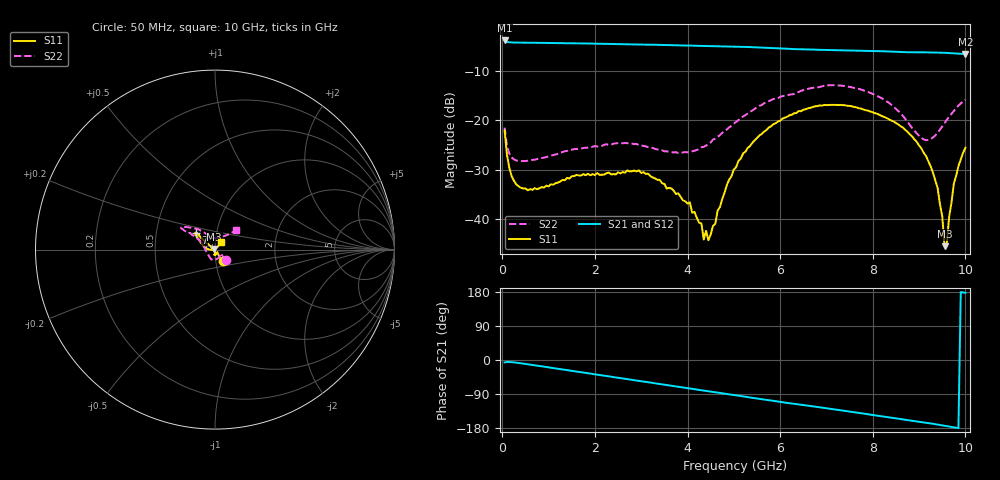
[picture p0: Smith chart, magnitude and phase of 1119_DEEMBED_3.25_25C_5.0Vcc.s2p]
!Hittite Microwave Corp.
!Digital Attenuator/PhaseShifter Rev 1.4.0
!Filename: C:\DATA\DATA\1119_DEEMBED_3.25_25C_5.0Vcc.s2p
!VNA ID: Agilent Technologies,N5224A,MY51441122,A.10.45.03
!Device type:
!2 Port Calibration.
!Temp(C): 25
!Lot Number:
!Serial Number:
!Operator:
!Misc:
!Attenuator:  3.250
# GHZ S DB R 50.0
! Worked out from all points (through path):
!   200 points, 50 MHz to 10 GHz, reference 50 ohm
!   highest |S21| = -3.90 dB at 50 MHz (marker M1); lowest = -6.7 dB at 10 GHz (marker M2)
!   group delay of S21, straight-line fit = 49.8 ps
!   lowest |S11| = -45.4 dB at 9.55 GHz (marker M3), VSWR 1.01, Z = 49.6 + j0.324 ohm
!   |S11| at or under -10 dB: start of sweep to end of sweep
!   |S22| runs from -28.3 to -12.9 dB; largest |S21 - S12| = 0.0015
!   S11 on the Smith chart (normalised r, x): 50 MHz: 1.08, -0.14; 7 GHz: 0.80, +0.15; 10 GHz: 1.07, +0.09
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0.05  -22.07 -57.0  -3.90 -6.4  -3.90 -6.4  -21.50 -43.9
0.1  -26.95 -59.6  -4.19 -5.2  -4.19 -5.2  -25.11 -40.8
0.2  -31.25 -54.2  -4.30 -5.7  -4.29 -5.7  -27.50 -33.4
0.4  -33.64 -48.9  -4.34 -8.6  -4.34 -8.6  -28.26 -31.3
1.75  -30.88 -89.8  -4.50 -33.3  -4.50 -33.4  -25.60 -74.2
3.4  -32.06 -93.4  -4.78 -63.4  -4.79 -63.4  -25.95 -130.0
4.05  -36.57 -91.4  -4.93 -75.2  -4.94 -75.3  -26.50 -162.4
4.35  -44.07 -117.4  -5.01 -80.6  -5.03 -80.7  -25.38 176.7
4.45  -44.24 -156.0  -5.04 -82.5  -5.06 -82.6  -24.70 171.8
5.05  -29.48 143.3  -5.16 -93.3  -5.17 -93.3  -20.33 149.7
5.75  -21.50 140.7  -5.39 -106.2  -5.41 -106.2  -16.16 147.0
6.7  -17.35 138.2  -5.73 -122.3  -5.74 -122.3  -13.47 147.6
7  -16.95 138.3  -5.82 -127.3  -5.83 -127.4  -12.97 147.1
8.35  -19.80 149.1  -6.12 -151.4  -6.12 -151.4  -16.51 130.2
8.85  -23.27 161.3  -6.29 -160.1  -6.29 -160.1  -21.59 115.5
9.25  -29.33 179.3  -6.31 -167.4  -6.33 -167.5  -23.79 85.4
9.400001  -33.67 -179.6  -6.34 -170.4  -6.35 -170.5  -22.55 67.6
9.5  -39.41 168.3  -6.37 -172.5  -6.39 -172.5  -21.26 58.3
9.55  -45.43 142.4  -6.39 -173.5  -6.41 -173.6  -20.56 54.8
9.6  -44.78 94.4  -6.42 -174.6  -6.43 -174.6  -19.90 51.9
9.75  -32.81 48.1  -6.50 -177.7  -6.51 -177.7  -18.13 46.2
10  -25.57 50.1  -6.65 177.3  -6.65 177.3  -15.86 42.8
